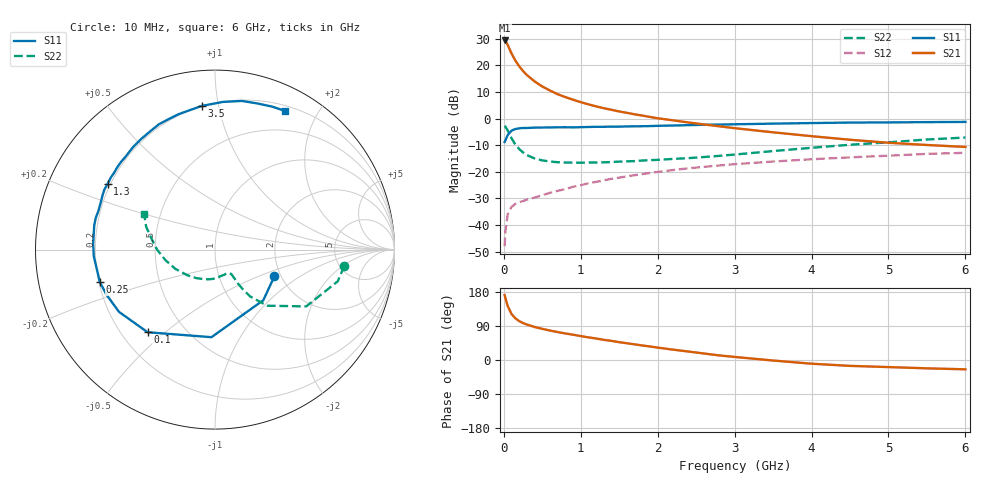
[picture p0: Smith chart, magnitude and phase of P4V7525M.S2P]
! SIEMENS Small Signal Semiconductors
! BFP182
! Si NPN RF Bipolar Junction Transistor in SOT143
! VCE = 0.75 V  IC = 25 mA
! Common Emitter S-Parameters:  March  1996
# GHz  S  MA  R  50
!  f  S11  S21  S12  S22
! GHz  MAG  ANG  MAG  ANG  MAG  ANG  MAG  ANG
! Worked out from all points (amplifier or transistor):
!   36 points, 10 MHz to 6 GHz, reference 50 ohm
!   highest |S21| = 29.4 dB at 10 MHz (marker M1)
!   |S21| within 3 dB of that: start of sweep to 70.5 MHz
!   unconditionally stable (mu >= 1): start of sweep to 19.5 MHz; 204.7 MHz to end of sweep
!   at 250 MHz: K = 1.15, MAG = 22.1 dB, |S12| = -31.0 dB
!   at 1.4 GHz: K = 2.24, MAG = 6.7 dB, |S12| = -22.6 dB
!   at 6 GHz: K = 1.77, MAG = -4.0 dB, |S12| = -12.9 dB
!   S11 on the Smith chart (normalised r, x): 10 MHz: 1.85, -0.63; 100 MHz: 0.31, -0.44; 250 MHz: 0.20, -0.13; 1.3 GHz: 0.19, +0.27; 3.5 GHz: 0.20, +0.89; 6 GHz: 0.26, +1.60
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0.01  0.3627 -24.3  29.41 171.5  0.004 74.4  0.7262 -7.2
0.02  0.3898 -46.3  28.77 163.5  0.0075 70.8  0.7062 -14.5
0.05  0.4884 -92.3  24.21 142.4  0.0158 59.0  0.5987 -31.9
0.1  0.5941 -129.2  16.75 121.4  0.0219 41.7  0.427 -47.1
0.15  0.6375 -147.0  12.32 109.9  0.0249 38.2  0.3254 -53.2
0.2  0.655 -157.5  9.615 102.6  0.0268 36.5  0.2675 -55.0
0.25  0.6669 -164.4  7.805 97.4  0.0282 37.0  0.2303 -55.9
0.3  0.6662 -169.2  6.573 93.5  0.03 38.7  0.2056 -56.0
0.4  0.6764 -176.8  5.002 87.1  0.0327 41.9  0.178 -56.1
0.5  0.6795 177.3  4.006 82.2  0.0363 43.6  0.1637 -56.4
0.6  0.6814 172.5  3.365 77.7  0.0403 46.5  0.1558 -57.8
0.7  0.6863 168.6  2.87 73.7  0.0438 48.0  0.1515 -59.9
0.9  0.6843 161.7  2.266 66.7  0.0523 50.8  0.1488 -64.1
1.1  0.6953 154.4  1.852 59.7  0.0608 51.7  0.1492 -70.1
1.3  0.7015 148.4  1.566 53.2  0.069 51.5  0.1506 -76.6
1.7  0.7163 136.7  1.202 41.3  0.0864 50.0  0.1588 -89.6
2.2  0.7408 123.9  0.927 27.3  0.108 46.4  0.1746 -108.2
2.8  0.7718 109.3  0.716 12.1  0.1314 40.4  0.1993 -130.4
3.5  0.8038 95.3  0.552 -1.4  0.1559 33.0  0.2454 -154.0
4.5  0.8416 79.8  0.4 -15.5  0.1867 22.7  0.3225 -179.9
5.5  0.8576 68.3  0.319 -22.0  0.2171 12.7  0.4043 161.6
6  0.8663 63.1  0.293 -24.6  0.2273 7.1  0.4402 153.6
